FUNCTION_BLOCK FB_DO_IED_LD1_LPHD1_PhyHealth EXTENDS FB_AcsiCommonDataClass
VAR_INPUT
	stVal: FB_AcsiDATypePhyHealth := (fc:=ACSI_FC_ST, TrgOp:=ACSI_TrgOp_dchg OR ACSI_TrgOp_dupd, bLinkResult:=THIS^.AddDataToContainer(ipData:=stVal));
	q: FB_AcsiDATypeQuality := (fc:=ACSI_FC_ST, TrgOp:=ACSI_TrgOp_qchg, bLinkResult:=THIS^.AddDataToContainer(ipData:=q));
	t: FB_AcsiDATypeTimeStamp := (fc:=ACSI_FC_ST, bLinkResult:=THIS^.AddDataToContainer(ipData:=t));
END_VAR
VAR
END_VAR

END_FUNCTION_BLOCK
